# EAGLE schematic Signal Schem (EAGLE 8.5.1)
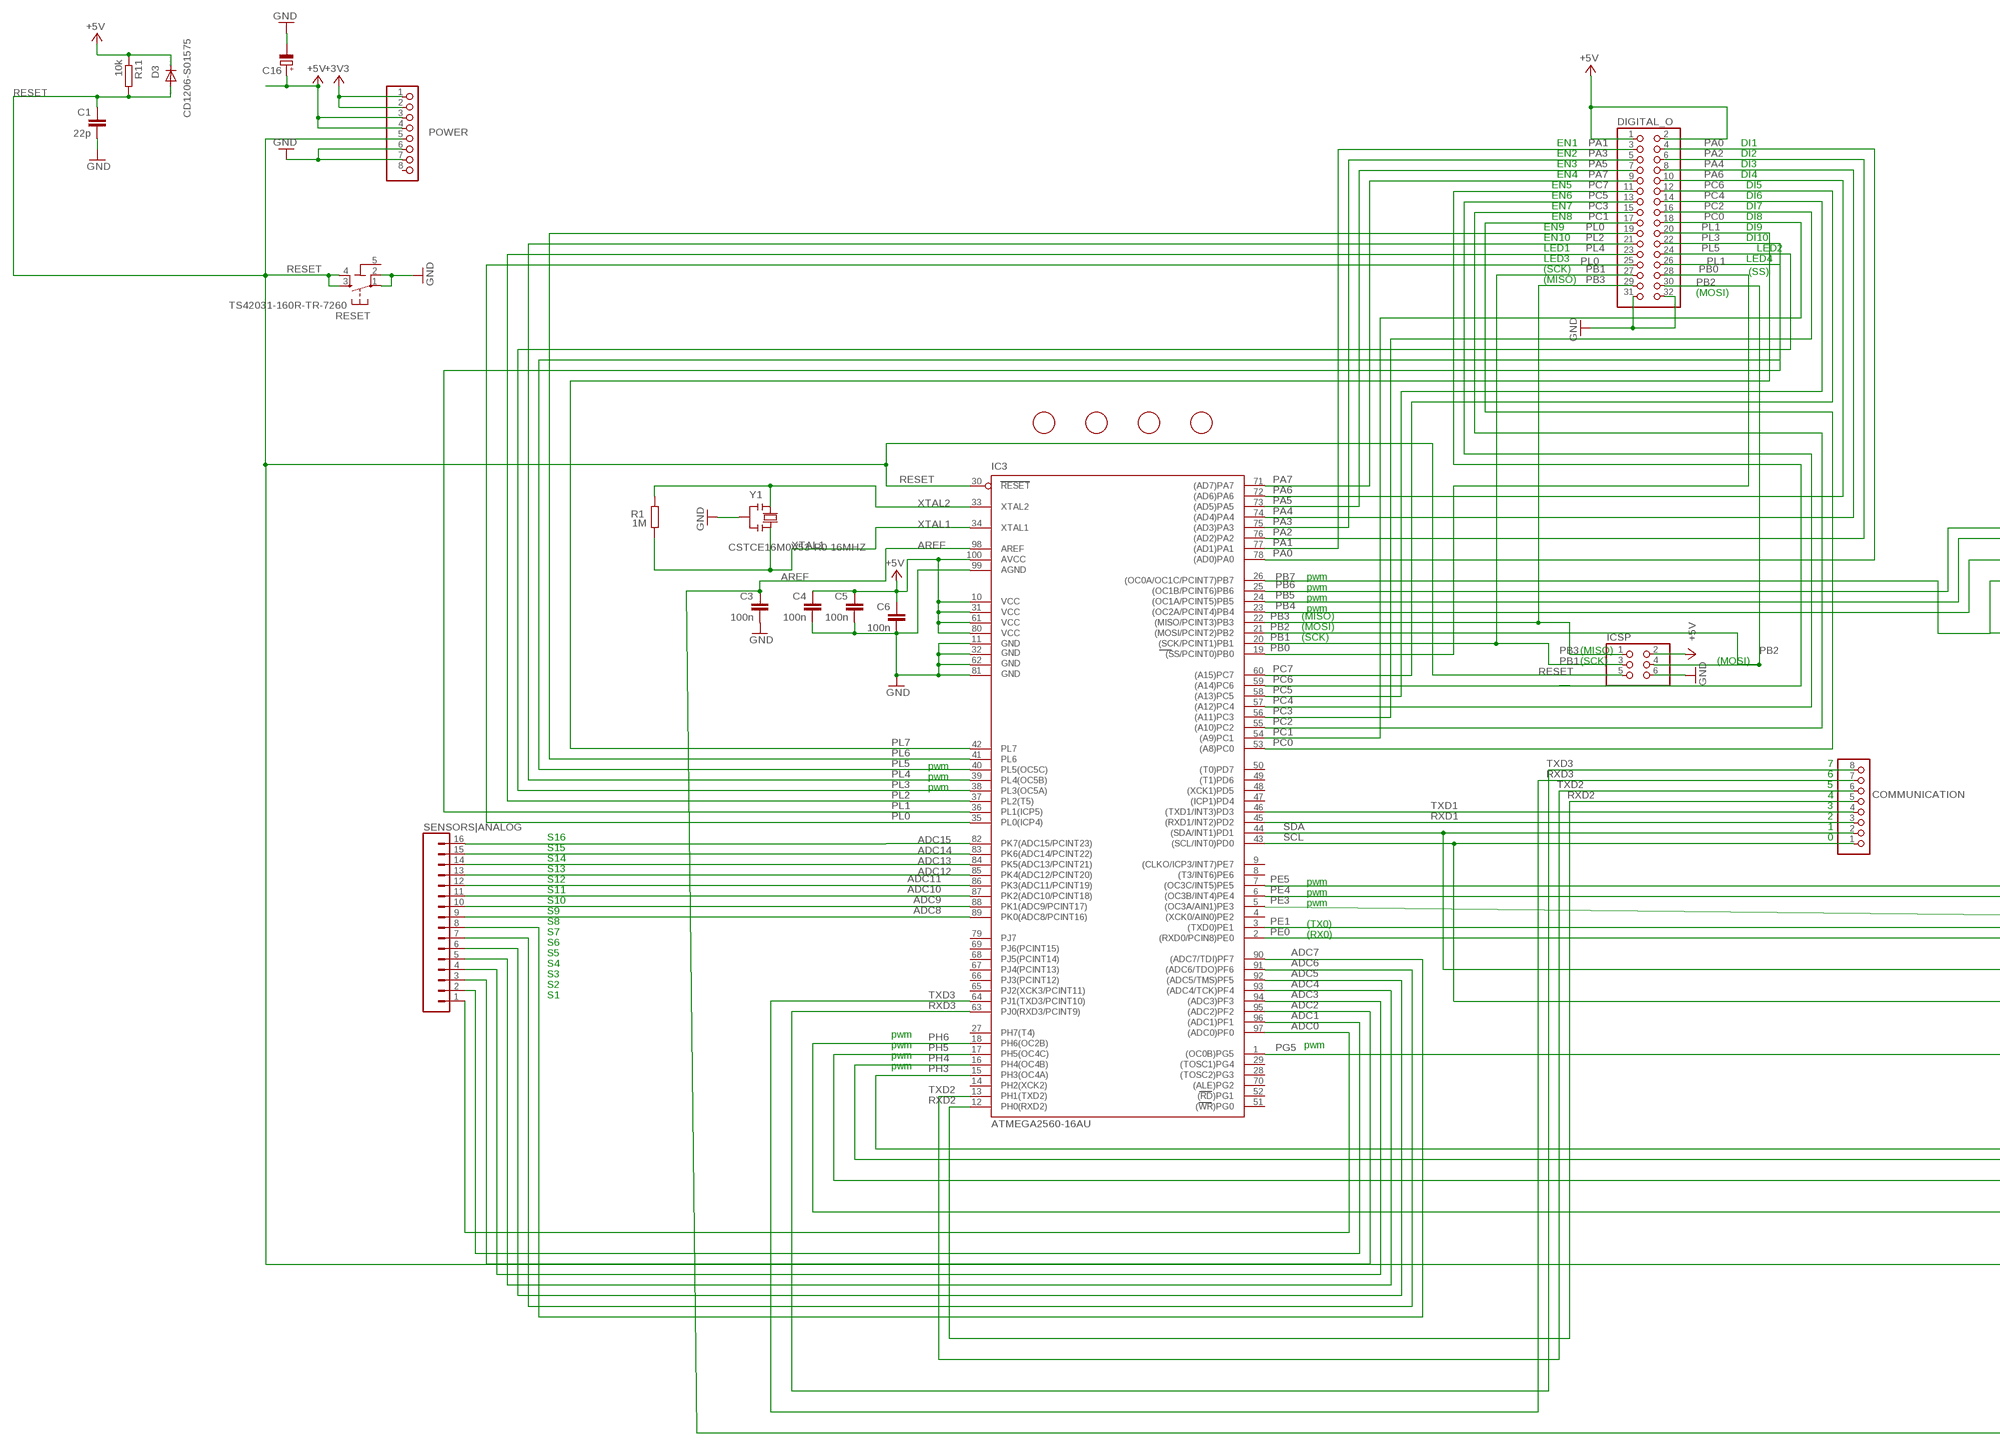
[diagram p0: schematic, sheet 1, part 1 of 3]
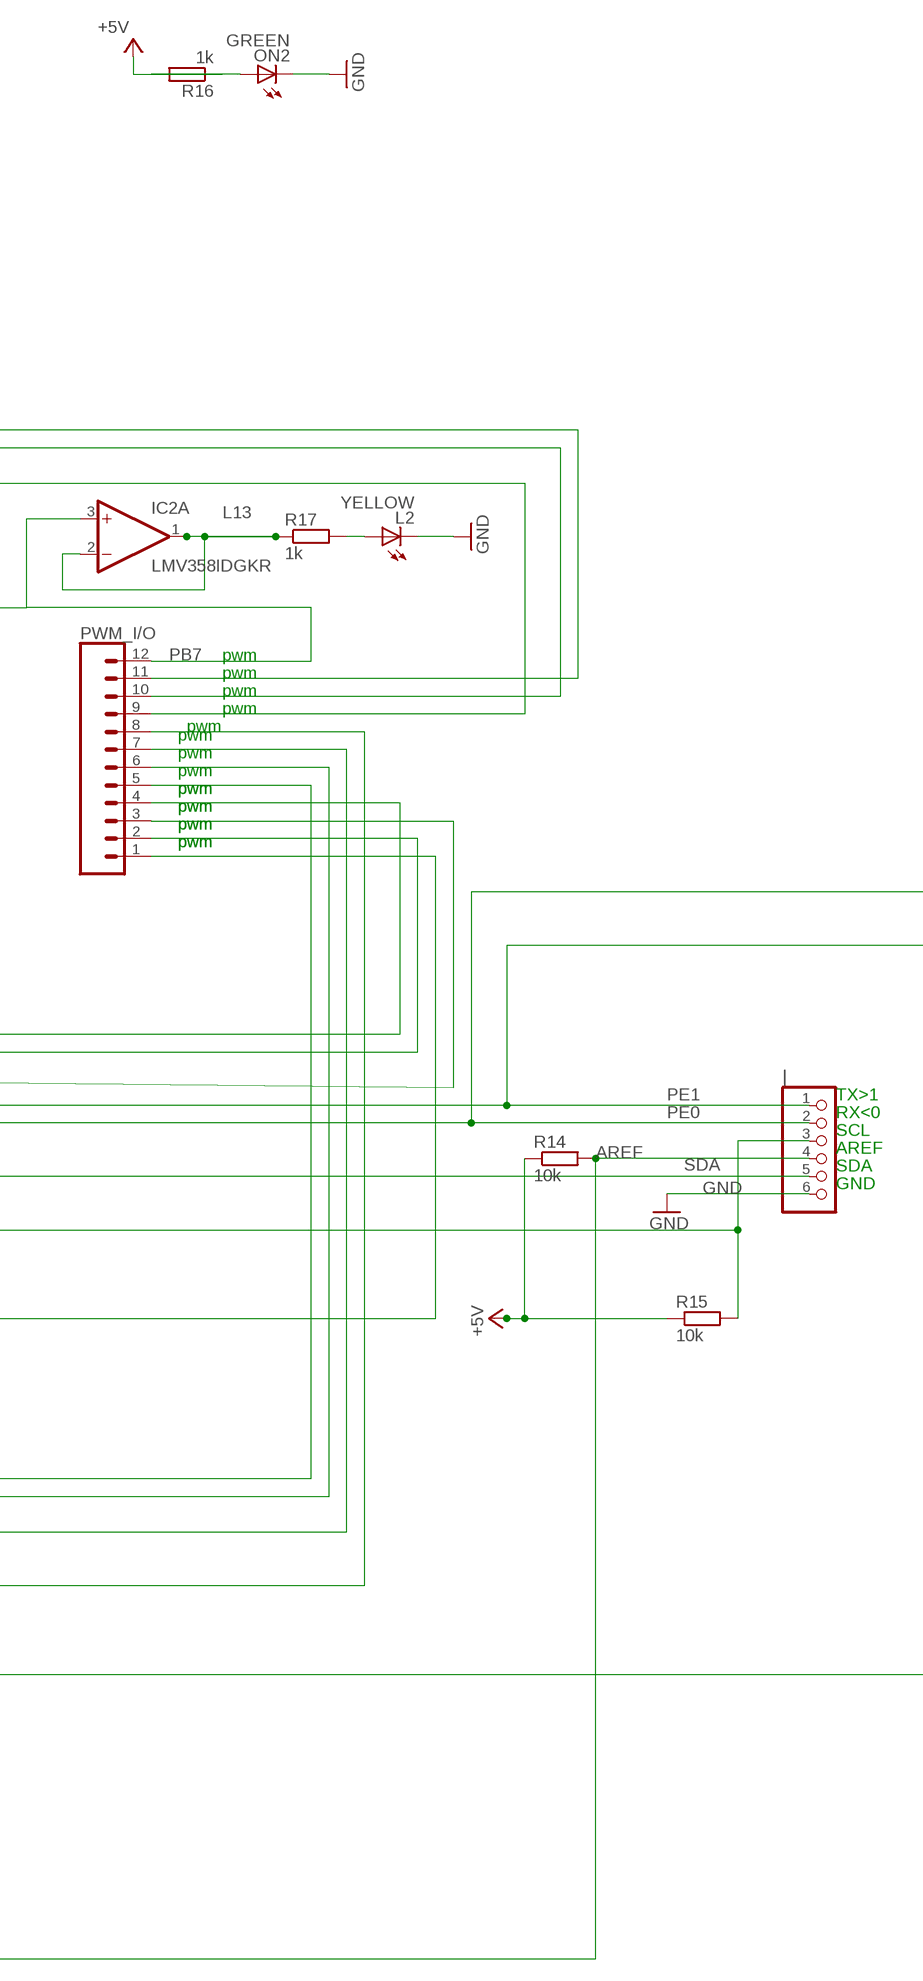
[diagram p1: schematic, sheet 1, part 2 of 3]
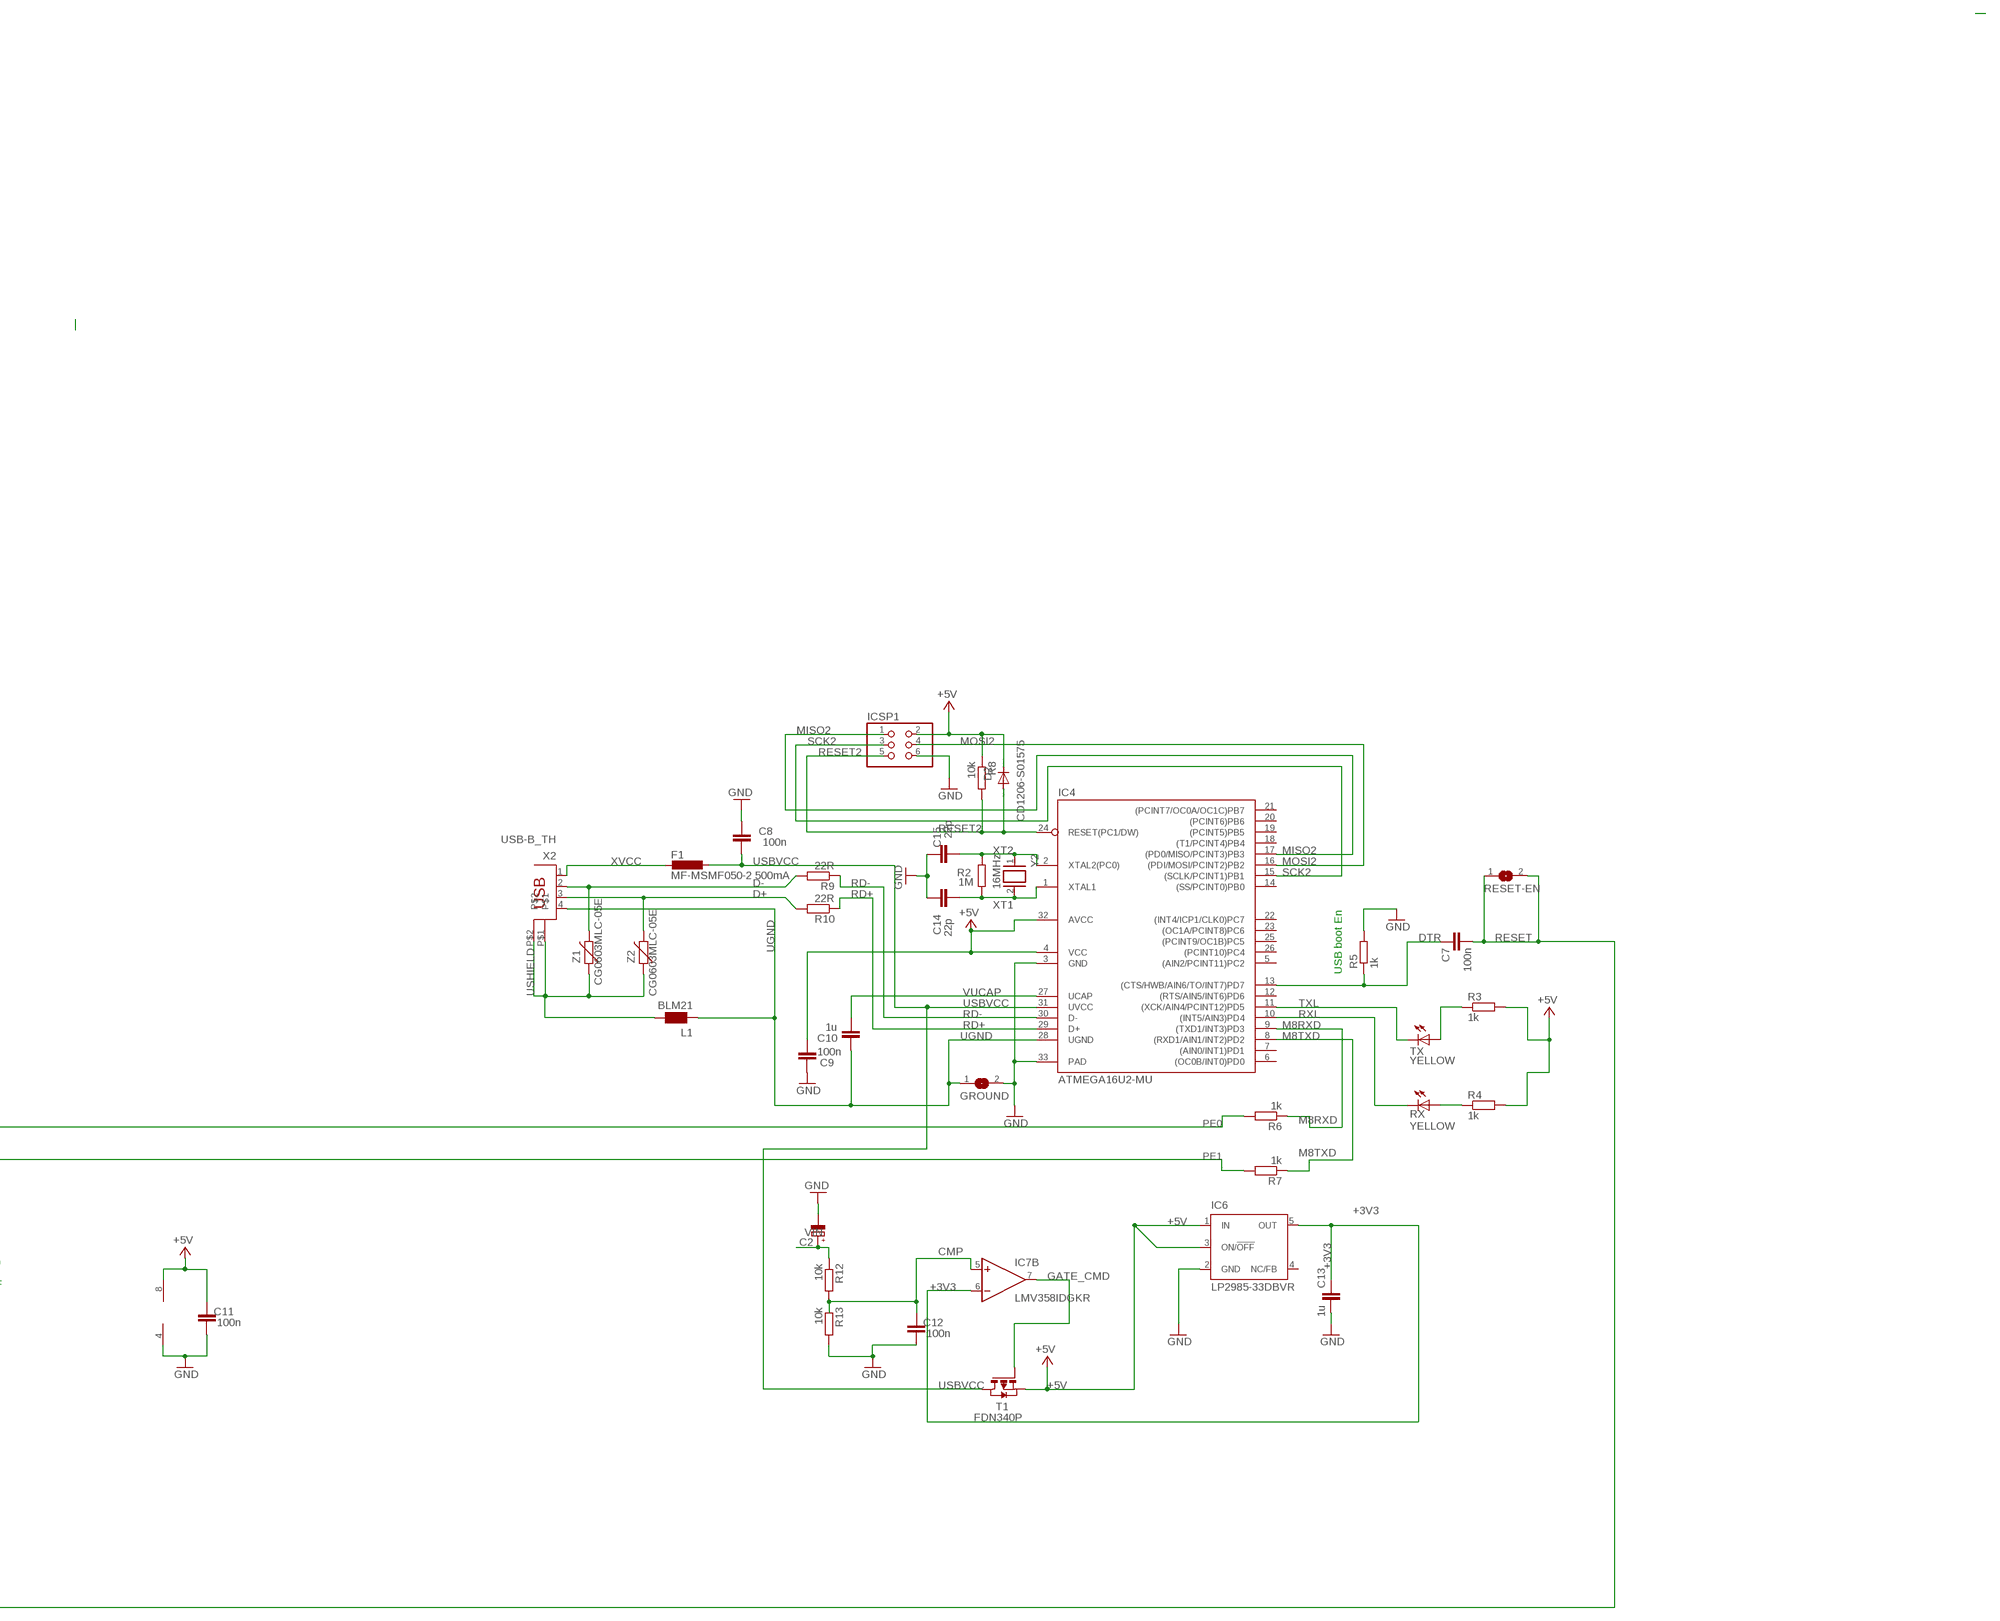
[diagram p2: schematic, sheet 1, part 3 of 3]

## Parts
C1  22p  C-EU0603-RND  [C0603-ROUND]
C2  CPOL-EUD  [PANASONIC_D]
C3  100n  C-EU0603-RND  [C0603-ROUND]
C4  100n  C-EU0603-RND  [C0603-ROUND]
C5  100n  C-EU0603-RND  [C0603-ROUND]
C6  100n  C-EU0603-RND  [C0603-ROUND]
C7  100n  C-EU0603-RND  [C0603-ROUND]
C8  100n  C-EU0603-RND  [C0603-ROUND]
C9  100n  C-EU0603-RND  [C0603-ROUND]
C10  1u  C-EU0603-RND  [C0603-ROUND]
C11  100n  C-EU0603-RND  [C0603-ROUND]
C12  100n  C-EU0603-RND  [C0603-ROUND]
C13  1u  C-EU0603-RND  [C0603-ROUND]
C14  22p  C-EU0603-RND  [C0603-ROUND]
C15  22p  C-EU0603-RND  [C0603-ROUND]
C16  CPOL-EUD  [PANASONIC_D]
COMMUNICATION  PINHD-1X8  [1X08]
D2  CD1206-S01575  DIODE-MINIMELF  [MINIMELF]
D3  CD1206-S01575  DIODE-MINIMELF  [MINIMELF]
DIGITAL_O  PINHD-2X16  [2X16]
F1  MF-MSMF050-2 500mA  L-EUL1812  [L1812]
FD1  FIDUCIALMOUNT  [FIDUCIA-MOUNT]
FD2  FIDUCIALMOUNT  [FIDUCIA-MOUNT]
FD3  FIDUCIALMOUNT  [FIDUCIA-MOUNT]
FD4  FIDUCIALMOUNT  [FIDUCIA-MOUNT]
GROUND  SJ  [SJ]
IC2  LMV358IDGKR  LMV358MMX  [MSOP08]
IC3  ATMEGA2560-16AU  ATMEGA25602560-16AU  [TQFP100]
IC4  ATMEGA16U2-MU  [MLF32]
IC6  LP2985-33DBVR  LP2985-XXDBVR33  [SOT23-DBV]
IC7  LMV358IDGKR  LMV358MMX  [MSOP08]
ICSP  PINHD-2X3  [2X03]
ICSP1  PINHD-2X3  [2X03]
L1  BLM21  WE-CBF_0805  [0805]
L2  YELLOW  LEDCHIP-LED0805  [CHIP-LED0805]
ON2  GREEN  LEDCHIP-LED0805  [CHIP-LED0805]
POWER  PINHD-1X8  [1X08]
PWM_I/O  CONN_12  [1X12]
R1  1M  R-EU_R0603  [R0603-ROUND]
R2  1M  R-EU_R0603  [R0603-ROUND]
R3  1k  R-EU_M1206  [M1206]
R4  1k  R-EU_M1206  [M1206]
R5  1k  R-EU_M1206  [M1206]
R6  1k  R-EU_M1206  [M1206]
R7  1k  R-EU_M1206  [M1206]
R8  10k  R-EU_M1206  [M1206]
R9  22R  R-EU_M1206  [M1206]
R10  22R  R-EU_M1206  [M1206]
R11  10k  R-EU_M1206  [M1206]
R12  10k  R-EU_M1206  [M1206]
R13  10k  R-EU_M1206  [M1206]
R14  10k  R-EU_M1206  [M1206]
R15  10k  R-EU_M1206  [M1206]
R16  1k  R-EU_M1206  [M1206]
R17  1k  R-EU_M1206  [M1206]
RESET  TS42031-160R-TR-7260  TS42  [TS42]
RESET-EN  SJ  [SJ]
RX  YELLOW  LEDCHIP-LED0805  [CHIP-LED0805]
SENSORS|ANALOG  CONN_16  [1X16]
T1  FDN340P  PMOSSOT23  [SOT-23]
TX  YELLOW  LEDCHIP-LED0805  [CHIP-LED0805]
X2  USB-B_TH  PN61729  [PN61729]
Y1  CSTCE16M0V53-R0 16MHZ  RESONATORMU  [RESONATOR]
Y2  16MHz  XTAL/S  [QS]
Z1  CG0603MLC-05E  VARISTORCN0603  [CT/CN0603]
Z2  CG0603MLC-05E  VARISTORCN0603  [CT/CN0603]
|  PINHD-1X6  [1X06]

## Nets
+3V3 [power]: C13.2 IC6.5(OUT) IC7.6(B:-IN) POWER.1 POWER.2
+5V [power usb]: C4.1 C5.1 C6.1 C9.1 C11.2 C16.+ D2.C D3.C DIGITAL_O.1 DIGITAL_O.2 IC3.10(VCC) IC3.31(VCC1) IC3.61(VCC2) IC3.80(VCC3) IC3.100(AVCC) IC4.4(VCC) IC4.32(AVCC) IC6.1(IN) IC6.3(ON/!OFF) IC7.8(P:V+) ICSP1.2 ICSP.2 POWER.3 POWER.4 R3.2 R4.2 R8.1 R11.1 R14.1 R15.1 R16.1 T1.2(S)
ADC0: IC3.97((ADC0)PF0) SENSORS|ANALOG.1
ADC1: IC3.96((ADC1)PF1) SENSORS|ANALOG.2
ADC2: IC3.95((ADC2)PF2) SENSORS|ANALOG.3
ADC3: IC3.94((ADC3)PF3) SENSORS|ANALOG.4
ADC4: IC3.93((ADC4/TCK)PF4) SENSORS|ANALOG.5
ADC5: IC3.92((ADC5/TMS)PF5) SENSORS|ANALOG.6
ADC6: IC3.91((ADC6/TDO)PF6) SENSORS|ANALOG.7
ADC7: IC3.90((ADC7/TDI)PF7) SENSORS|ANALOG.8
ADC8: IC3.89(PK0(ADC8/PCINT16)) SENSORS|ANALOG.9
ADC9: IC3.88(PK1(ADC9/PCINT17)) SENSORS|ANALOG.10
ADC10: IC3.87(PK2(ADC10/PCINT18)) SENSORS|ANALOG.11
ADC11: IC3.86(PK3(ADC11/PCINT19)) SENSORS|ANALOG.12
ADC12: IC3.85(PK4(ADC12/PCINT20)) SENSORS|ANALOG.13
ADC13: IC3.84(PK5(ADC13/PCINT21)) SENSORS|ANALOG.14
ADC14: IC3.83(PK6(ADC14/PCINT22)) SENSORS|ANALOG.15
ADC15: IC3.82(PK7(ADC15/PCINT23)) SENSORS|ANALOG.16
AREF: C3.1 IC3.98(AREF) R14.2 |.4
CMP: C12.2 IC7.5(B:+IN) R12.2 R13.1
D+: R10.2 X2.3 Z2.2
D-: R9.2 X2.2 Z1.2
DTR: C7.1 IC4.13((CTS/HWB/AIN6/TO/INT7)PD7) R5.1
GATE_CMD: IC7.7(B:OUT) T1.3(G)
GND [gnd]: C1.2 C2.- C3.2 C4.2 C5.2 C6.2 C8.2 C9.2 C11.1 C12.1 C13.1 C14.2 C15.2 C16.- DIGITAL_O.31 DIGITAL_O.32 GROUND.2 IC3.11(GND) IC3.32(GND1) IC3.62(GND2) IC3.81(GND3) IC3.99(AGND) IC4.3(GND) IC4.33(PAD) IC6.2(GND) IC7.4(P:V-) ICSP1.6 ICSP.6 L2.C ON2.C POWER.6 POWER.7 R5.2 R13.2 RESET.1 RESET.2 Y1.2 |.6
L13: IC2.1(A:OUT) IC2.2(A:-IN) R17.1
M8RXD: IC4.9((TXD1/INT3)PD3) R6.1
M8TXD: IC4.8((RXD1/AIN1/INT2)PD2) R7.1
MISO2: IC4.17((PD0/MISO/PCINT3)PB3) ICSP1.1
MOSI2: IC4.16((PDI/MOSI/PCINT2)PB2) ICSP1.4
N$10: L2.A R17.2
N$11: ON2.A R16.2
N$54: R4.1 RX.A
N$55: R3.1 TX.A
PA0: DIGITAL_O.4 IC3.78((AD0)PA0)
PA1: DIGITAL_O.3 IC3.77((AD1)PA1)
PA2: DIGITAL_O.6 IC3.76((AD2)PA2)
PA3: DIGITAL_O.5 IC3.75((AD3)PA3)
PA4: DIGITAL_O.8 IC3.74((AD4)PA4)
PA5: DIGITAL_O.7 IC3.73((AD5)PA5)
PA6: DIGITAL_O.10 IC3.72((AD6)PA6)
PA7: DIGITAL_O.9 IC3.71((AD7)PA7)
PB0: DIGITAL_O.28 IC3.19((SS/PCINT0)PB0)
PB1: DIGITAL_O.27 IC3.20((SCK/PCINT1)PB1) ICSP.3
PB2: DIGITAL_O.30 IC3.21((MOSI/PCINT2)PB2) ICSP.4
PB3: DIGITAL_O.29 IC3.22((MISO/PCINT3)PB3) ICSP.1
PB4: IC3.23((OC2A/PCINT4)PB4) PWM_I/O.9
PB5: IC3.24((OC1A/PCINT5)PB5) PWM_I/O.10
PB6: IC3.25((OC1B/PCINT6)PB6) PWM_I/O.11
PB7: IC2.3(A:+IN) IC3.26((OC0A/OC1C/PCINT7)PB7) PWM_I/O.12
PC0: DIGITAL_O.17 IC3.53((A8)PC0)
PC1: DIGITAL_O.18 IC3.54((A9)PC1)
PC2: DIGITAL_O.15 IC3.55((A10)PC2)
PC3: DIGITAL_O.16 IC3.56((A11)PC3)
PC4: DIGITAL_O.13 IC3.57((A12)PC4)
PC5: DIGITAL_O.14 IC3.58((A13)PC5)
PC6: DIGITAL_O.11 IC3.59((A14)PC6)
PC7: DIGITAL_O.12 IC3.60((A15)PC7)
PE0: IC3.2((RXD0/PCIN8)PE0) R6.2 |.2
PE1: IC3.3((TXD0)PE1) R7.2 |.1
PE3: IC3.5((OC3A/AIN1)PE3) PWM_I/O.3
PE4: IC3.6((OC3B/INT4)PE4) PWM_I/O.2
PE5: IC3.7((OC3C/INT5)PE5) PWM_I/O.4
PG5: IC3.1((OC0B)PG5) PWM_I/O.1
PH3: IC3.15(PH3(OC4A)) PWM_I/O.5
PH4: IC3.16(PH4(OC4B)) PWM_I/O.6
PH5: IC3.17(PH5(OC4C)) PWM_I/O.7
PH6: IC3.18(PH6(OC2B)) PWM_I/O.8
PL0: DIGITAL_O.25 IC3.35(PL0(ICP4))
PL1: DIGITAL_O.26 IC3.36(PL1(ICP5))
PL2: DIGITAL_O.23 IC3.37(PL2(T5))
PL3: DIGITAL_O.24 IC3.38(PL3(OC5A))
PL4: DIGITAL_O.21 IC3.39(PL4(OC5B))
PL5: DIGITAL_O.22 IC3.40(PL5(OC5C))
PL6: DIGITAL_O.19 IC3.41(PL6)
PL7: DIGITAL_O.20 IC3.42(PL7)
RD+: IC4.29(D+) R10.1
RD-: IC4.30(D-) R9.1
RESET: C1.1 C7.2 D3.A IC3.30(RESET) ICSP.5 POWER.5 R11.2 RESET-EN.1 RESET-EN.2 RESET.3 RESET.4
RESET2: D2.A IC4.24(RESET(PC1/DW)) ICSP1.5 R8.2
RXD1: COMMUNICATION.3 IC3.45((RXD1/INT2)PD2)
RXD2: COMMUNICATION.5 IC3.12(PH0(RXD2))
RXD3: COMMUNICATION.8 IC3.63(PJ0(RXD3/PCINT9))
RXL: IC4.10((INT5/AIN3)PD4) RX.C
SCK2: IC4.15((SCLK/PCINT1)PB1) ICSP1.3
SCL: COMMUNICATION.1 IC3.43((SCL/INT0)PD0) R15.2 |.3
SDA: COMMUNICATION.2 IC3.44((SDA/INT1)PD1) |.5
TXD1: COMMUNICATION.4 IC3.46((TXD1/INT3)PD3)
TXD2: COMMUNICATION.6 IC3.13(PH1(TXD2))
TXD3: COMMUNICATION.7 IC3.64(PJ1(TXD3/PCINT10))
TXL: IC4.11((XCK/AIN4/PCINT12)PD5) TX.C
UGND [gnd]: C10.2 GROUND.1 IC4.28(UGND) L1.1 X2.4
USBVCC [power usb]: C8.1 F1.1 IC4.31(UVCC) T1.1(D)
USHIELD [gnd]: L1.2 X2.P$1 X2.P$2 Z1.1 Z2.1
VIN [power]: C2.+ R12.1
VUCAP: C10.1 IC4.27(UCAP)
XT1: C14.1 IC4.1(XTAL1) R2.1 Y2.2
XT2: C15.1 IC4.2(XTAL2(PC0)) R2.2 Y2.1
XTAL1: IC3.34(XTAL1) R1.1 Y1.3
XTAL2: IC3.33(XTAL2) R1.2 Y1.1
XVCC [power usb]: F1.2 X2.1
Unconnected: IC2.5(B:+IN) IC2.6(B:-IN) IC2.7(B:OUT) IC3.4((XCK0/AIN0)PE2) IC3.8((T3/INT6)PE6) IC3.9((CLKO/ICP3/INT7)PE7) IC3.14(PH2(XCK2)) IC3.27(PH7(T4)) IC3.28((TOSC2)PG3) IC3.29((TOSC1)PG4) IC3.47((ICP1)PD4) IC3.48((XCK1)PD5) IC3.49((T1)PD6) IC3.50((T0)PD7) IC3.51((WR)PG0) IC3.52((RD)PG1) IC3.65(PJ2(XCK3/PCINT11)) IC3.66(PJ3(PCINT12)) IC3.67(PJ4(PCINT13)) IC3.68(PJ5(PCINT14)) IC3.69(PJ6(PCINT15)) IC3.70((ALE)PG2) IC3.79(PJ7) IC4.5((AIN2/PCINT11)PC2) IC4.6((OC0B/INT0)PD0) IC4.7((AIN0/INT1)PD1) IC4.12((RTS/AIN5/INT6)PD6) IC4.14((SS/PCINT0)PB0) IC4.18((T1/PCINT4)PB4) IC4.19((PCINT5)PB5) IC4.20((PCINT6)PB6) IC4.21((PCINT7/OC0A/OC1C)PB7) IC4.22((INT4/ICP1/CLK0)PC7) IC4.23((OC1A/PCINT8)PC6) IC4.25((PCINT9/OC1B)PC5) IC4.26((PCINT10)PC4) IC6.4(NC/FB) IC7.1(A:OUT) IC7.2(A:-IN) IC7.3(A:+IN) POWER.8

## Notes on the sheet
- EN1 | DI1
- EN2 | DI2
- EN3 | DI3
- EN4 | DI4
- EN5 | DI5
- EN6 | DI6
- EN7 | DI7
- EN8 | DI8
- EN9 | DI9
- EN10 | DI10
- LED1 | LED2
- LED3 | LED4
- (SCK) | (SS)
- (MISO)
- (MOSI)
- pwm
- pwm
- pwm
- pwm
- (MISO)
- (MOSI)
- (SCK)
- (MISO) | USB boot En
- (SCK) | (MOSI) | pwm
- pwm
- pwm
- pwm
- pwm
- pwm
- pwm
- pwm
- pwm | pwm
- pwm | pwm
- 7 | pwm | pwm
- pwm
- 6 | pwm | pwm
- pwm
- pwm | 5
- 4
- 3
- 2
- 1
- S16 | 0
- S15
- S14
- S13
- S12 | pwm
- S11 | pwm
- S10 | pwm
- S9
- S8 | (TX0) | TX>1
- S7 | (RX0) | RX<0
- S6 | SCL
- S5 | AREF
- S4 | SDA
- S3 | GND
- S2
- S1
- pwm
- pwm | pwm
- pwm
- pwm

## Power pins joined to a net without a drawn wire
5-GND: RESET.5(5-GND)
V+: IC2.8(P:V+)
V-: IC2.4(P:V-)

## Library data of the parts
C1 C3-C15 = SmartPrj:C-EU: CAPACITOR, European symbol
C2 C16 = rcl:CPOL-EU: POLARIZED CAPACITOR, European symbol; SPICEPREFIX: C
COMMUNICATION POWER = SmartPrj:PINHD-1X8: PIN HEADER
D2 D3 = diode:DIODE-: DIODE
DIGITAL_O = pinhead:PINHD-2X16: PIN HEADER
F1 = rcl:L-EU: INDUCTOR, European symbol
FD1-FD4 = SmartPrj:FIDUCIALMOUNT
GROUND RESET-EN = jumper:SJ: SMD solder JUMPER
IC2 IC7 = linear:LMV358?*: Dual General Purpose, Low Voltage, Rail-to-Rail Output Operational Amplifiers Source: http://www.national.com/mpf/LM/LMV321.html http://www.national.com/dt/lmv_qual.pdf
IC3 = SmartPrj:ATMEGA2560: MICROCONTROLLER 64/128/256 Kbytes FLASH 4 Kbytes EEPROM 8 Kbytes SRAM 86 General Purpose I/O pins 12-channels16-bit PWM 4 x Serial USARTs 16-channels 10-bit A/D
IC4 = SmartPrj:ATMEGA16U2-
IC6 = SmartPrj:LP2985-XXDBVR: ULTRALOW-POWER 50-mA LOW-DROPOUT LINEAR REGULATORS 50-mA Low-Dropout Regulator Source: http://focus.ti.com/lit/ds/symlink/tps77001.pdf
ICSP ICSP1 = SmartPrj:PINHD-2X3: PIN HEADER
L1 = wuerth-elektronik:WE-CBF: SMD EMI Suppression Ferrite Beads
L2 ON2 RX TX = led:LED: LED
PWM_I/O = SparkFun-Connectors:CONN_12: Multi connection point. Often used as Generic Header-pin footprint for 0.1 inch spaced/style header connections On any of the 0.1 inch spaced packages, you can populate with these: Break Away Headers - Straight (PRT-00116) Break Away Male Headers - Right Angle (PRT-00553) Female Headers (PRT-00115)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
R1 R2 = SmartPrj:R-EU_: RESISTOR, European symbol
R3-R17 = rcl:R-EU_: RESISTOR, European symbol; SPICEPREFIX: R
RESET = SmartPrj:TS42: TS42 Dongnan Electronics Tact switch VDC 12V - 50mA
SENSORS|ANALOG = SparkFun-Connectors:CONN_16: Multi connection point. Often used as Generic Header-pin footprint for 0.1 inch spaced/style header connections On any of the 0.1 inch spaced packages, you can populate with these: Break Away Headers - Straight (PRT-00116) Break Away Male Headers - Right Angle (PRT-00553) Female Headers (PRT-00115)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
T1 = zetex:PMOSSOT23: MOS FET; OC_FARNELL: unknown; OC_NEWARK: unknown
X2 = SmartPrj:PN61729: BERG USB connector
Y1 = SmartPrj:RESONATOR
Y2 = SmartPrj:XTAL/S: CRYSTAL
Z1 Z2 = varistor:VARISTOR: VARISTOR
| = pinhead:PINHD-1X6: PIN HEADER

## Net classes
0 default: width 0.203 mm, drill 0.406 mm, clearance 0.203 mm
1 power: width 0.61 mm, drill 0.406 mm, clearance 0.203 mm
2 gnd: width 0.305 mm, drill 0.406 mm, clearance 0.203 mm
3 power usb: width 0.508 mm, drill 0.406 mm, clearance 0.203 mm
